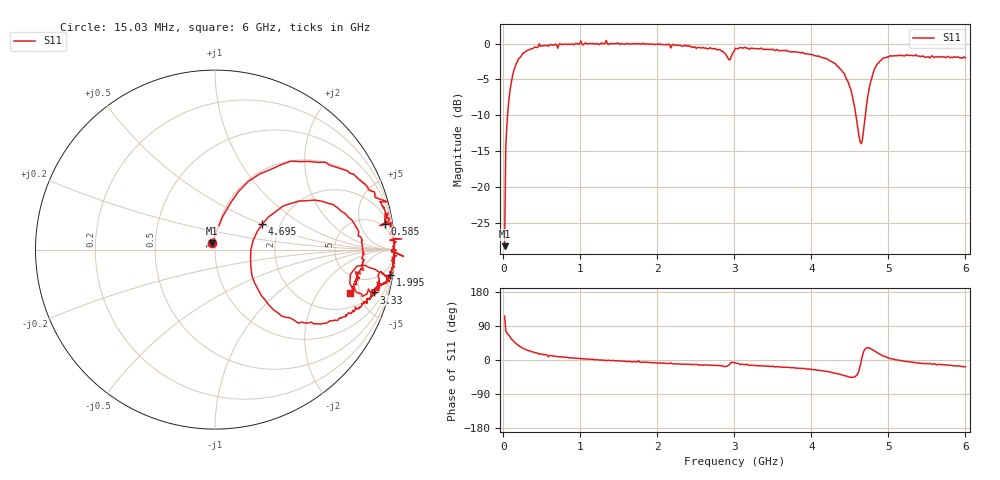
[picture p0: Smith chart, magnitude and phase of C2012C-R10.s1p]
!	Network	Analyzer	HP8753E.07.74:	Oct	30	2002	Serial	No.	JP38451487
!	Hewlett-Packard
!	7	Sep	2009	12:12:40
!	Frequency	S11
#	HZ	S	RI	R	50
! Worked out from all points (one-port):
!   400 points, 15.03 MHz to 6 GHz, reference 50 ohm
!   lowest |S11| = -28.3 dB at 15.03 MHz (marker M1), VSWR 1.08, Z = 48.2 + j3.34 ohm
!   |S11| at or under -10 dB: start of sweep to 53.7 MHz; 4.578 GHz to 4.701 GHz (122.9 MHz wide, 2.65 % of centre)
!   S11 on the Smith chart (normalised r, x): 15.03 MHz: 0.96, +0.07; 585 MHz: 4, +12; 1.995 GHz: 1, -14; 3.33 GHz: 2.23, -6.84; 4.695 GHz: 1.62, +0.50; 6 GHz: 3.11, -4.06
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1.502992e7  -0.0168 0.0346
3.002985e7  0.0415 0.182
6.00297e7  0.133 0.326
1.200294e8  0.368 0.473
1.95029e8  0.613 0.487
3.150284e8  0.813 0.382
4.650277e8  0.961 0.266
5.550272e8  0.938 0.24
5.850271e8  0.947 0.142
7.650262e8  0.971 0.144
1.335023e9  1.05 -0.0378
1.515022e9  0.986 -0.0433
1.99502e9  0.977 -0.143
2.265019e9  0.959 -0.173
2.805016e9  0.878 -0.226
2.925015e9  0.751 -0.189
2.955015e9  0.791 -0.0924
3.015015e9  0.917 -0.127
3.330013e9  0.887 -0.239
3.765011e9  0.821 -0.301
4.215009e9  0.669 -0.392
4.515007e9  0.329 -0.338
4.635007e9  0.198 -0.0495
4.695007e9  0.263 0.141
4.800006e9  0.554 0.276
4.935005e9  0.78 0.137
5.265004e9  0.824 -0.0689
6e9  0.754 -0.243
